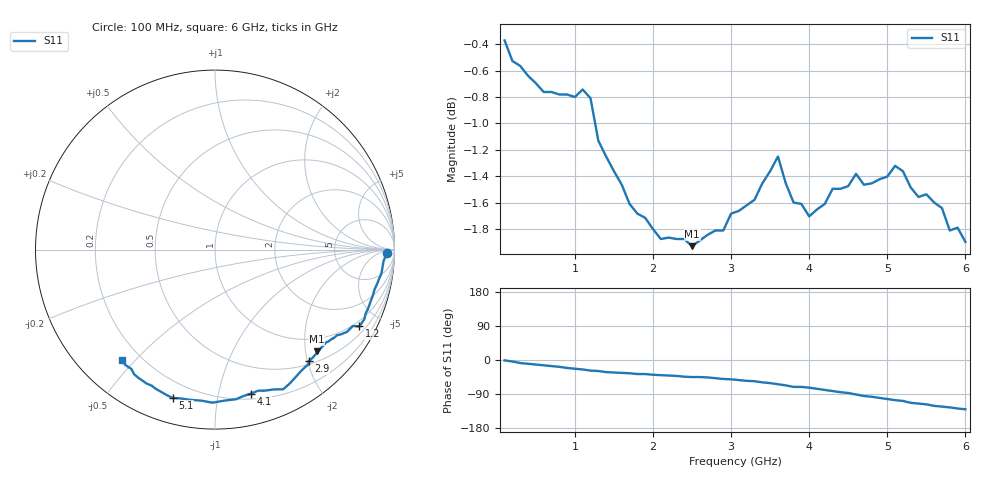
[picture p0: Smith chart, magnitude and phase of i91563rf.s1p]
!  IAM-91563  Typical Reflection Coefficients, RF port
!  Tc=25 C, Vdd= 3 V
!  LAST UPDATED 02-25-97
# ghz s ma r 50
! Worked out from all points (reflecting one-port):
!   60 points, 100 MHz to 6 GHz, reference 50 ohm
!   lowest |S11| = -1.9 dB at 2.5 GHz (marker M1), VSWR 9.05, Z = 35.2 - j111 ohm
!   phase of S11 starts at -1 deg and turns -129 deg over the sweep
!   S11 on the Smith chart (normalised r, x): 100 MHz: 40, -16; 1.2 GHz: 0.77, -3.87; 2.9 GHz: 0.55, -2.02; 4.1 GHz: 0.25, -1.25; 5.1 GHz: 0.12, -0.75; 6 GHz: 0.13, -0.46
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0.1  0.958 -1.0
0.3  0.937 -8.0
0.9  0.914 -21.0
1.2  0.911 -28.0
1.3  0.878 -29.0
1.4  0.866 -32.0
1.6  0.845 -34.0
1.8  0.824 -37.0
2.4  0.806 -44.0
2.5  0.801 -45.0
2.7  0.809 -46.0
2.9  0.812 -50.0
3.1  0.826 -53.0
3.3  0.834 -56.0
3.5  0.855 -61.0
3.6  0.866 -64.0
3.8  0.832 -71.0
3.9  0.831 -71.0
4.1  0.827 -76.0
4.5  0.844 -87.0
4.6  0.853 -91.0
4.7  0.845 -95.0
5.1  0.859 -106.0
5.2  0.855 -108.0
5.3  0.843 -113.0
5.5  0.838 -117.0
5.6  0.832 -121.0
6  0.804 -130.0
